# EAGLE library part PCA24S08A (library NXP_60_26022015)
1024 × 8-bit CMOS EEPROM with access protection The PCA24S08A provides 8192 bits of serial Electrically Erasable and Programmable Read-Only Memory (EEPROM) organized as 1024 words of 8 bits each. Data bytes are received and transmitted via the serial I2 C-bus. Access permissions limiting reads or writes are set via the I2 C-bus to isolate blocks of memory from improper access. The PCA24S08A is intended to be pin compatible with standard 24C08 serial EEPROM devices except for pins 1, 2, and 3, which are address pins in the standard part. Other exceptions to the PCA24S08A serial EEPROM data sheet are noted in Section 6.6. All bits are sent to or read from the device, most significant bit first, in a manner consistent with the 24C08 serial EEPROM. The bit fields in this document are correspondingly listed with the MSB on the left and the LSB on the right. The EEPROM memory is broken up into 8 blocks of 1 kbit (128 bytes) each. Within each block, the memory is physically organized in to 8 pages of 128 bits (16 bytes) each. In addition to these 8 kbits, there are two more 128-bit pages that are used to store the access protection and ID information. There are a total of 8448 bits of EEPROM memory available in the PCA24S08A. Access protection (both read and write) is organized on a block basis for block 1 through block 7 and on a page and a block basis for block 0. Protection information for these blocks and pages is stored in one of the additional pages of EEPROM memory that is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
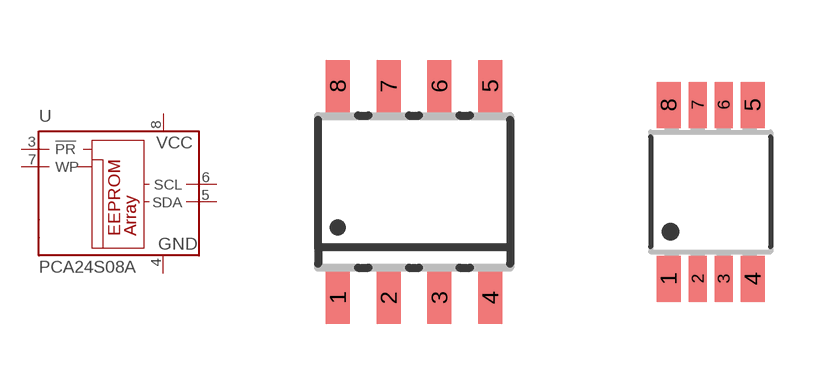
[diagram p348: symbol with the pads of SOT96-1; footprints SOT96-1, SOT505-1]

Designator prefix U

## PCA24S08AD  [SOT96-1]
3  !PR!
4  GND  pwr
5  SDA
6  SCL  in
7  WP  in
8  VCC  pwr

## PCA24S08ADP  [SOT505-1]
Pads as for SOT96-1

## Footprint SOT96-1 (pad centres in mm)
SOT96-1 SO8: plastic small outline package; 8 leads; body width 3.9 mm JEDEC: MS-012 IEC: 076E03
smd 0.6 x 1.3: 1 -1.905,-2.65; 2 -0.635,-2.65; 3 0.635,-2.65; 4 1.905,-2.65; 5 1.905,2.65; 6 0.635,2.65; 7 -0.635,2.65; 8 -1.905,2.65

## Footprint SOT505-1 (pad centres in mm)
SOT505-1 TSSOP8: plastic thin shrink small outline package; 8 leads; body width 3 mm JEDEC: -- IEC: --
smd 0.6 x 1.15: 1 -1.05,-2.175; 4 1.05,-2.175; 5 1.05,2.175; 8 -1.05,2.175
smd 0.45 x 1.15: 2 -0.325,-2.175; 3 0.325,-2.175; 6 0.325,2.175; 7 -0.325,2.175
